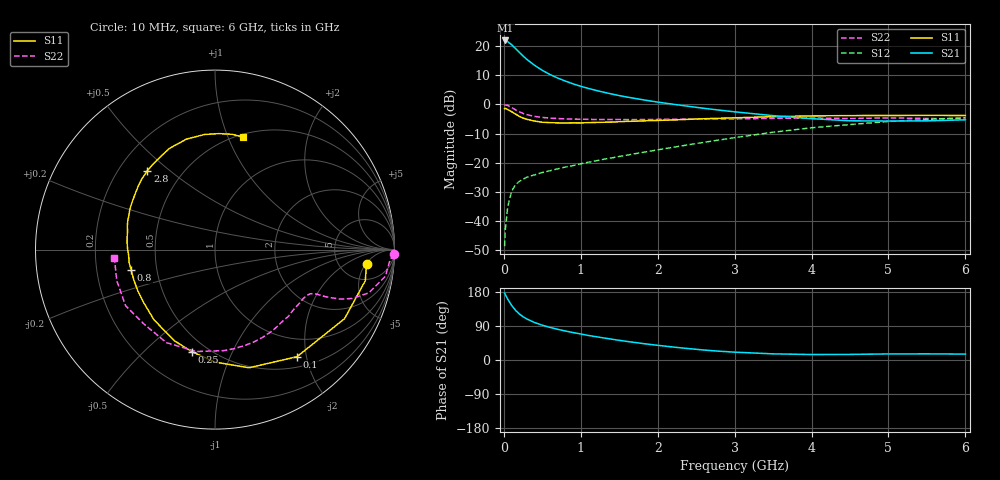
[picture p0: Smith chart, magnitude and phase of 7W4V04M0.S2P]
! Infineon Technologies  Discrete & RF Semiconductors
! BFS17W
! Si NPN RF Bipolar Junction Transistor in SOT323
! VCE = 4 V  IC = 4 mA
! Common Emitter S-Parameters:  August  1999
# GHz  S  MA  R  50
!  f  S11  S21  S12  S22
! GHz  MAG  ANG  MAG  ANG  MAG  ANG  MAG  ANG
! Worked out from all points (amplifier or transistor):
!   36 points, 10 MHz to 6 GHz, reference 50 ohm
!   highest |S21| = 22.0 dB at 20 MHz (marker M1)
!   |S21| within 3 dB of that: start of sweep to 160.8 MHz
!   unconditionally stable (mu >= 1): 623.7 MHz to 2.79 GHz; 4.312 GHz to end of sweep
!   at 250 MHz: K = 0.53, MSG = 21.1 dB, |S12| = -25.6 dB
!   at 1.4 GHz: K = 1.26, MAG = 7.9 dB, |S12| = -18.4 dB
!   at 6 GHz: K = 1.08, MAG = -2.1 dB, |S12| = -4.5 dB
!   S11 on the Smith chart (normalised r, x): 10 MHz: 9, -5; 100 MHz: 0.67, -1.83; 250 MHz: 0.41, -0.71; 800 MHz: 0.36, -0.11; 2.8 GHz: 0.32, +0.42; 6 GHz: 0.53, +1.13
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0.01  0.8485 -5.6  12.51 176.6  0.0037 87.1  0.9965 -1.4
0.02  0.8551 -11.7  12.53 172.1  0.0073 90.6  0.976 -3.7
0.05  0.8179 -28.1  11.97 160.7  0.0174 77.3  0.9611 -8.9
0.1  0.7513 -52.6  10.64 144.6  0.032 65.6  0.8906 -15.7
0.15  0.6852 -73.9  9.169 131.4  0.0418 56.2  0.8113 -19.6
0.2  0.6269 -90.0  7.874 121.7  0.0477 52.4  0.7494 -21.6
0.25  0.583 -102.9  6.773 114.2  0.0522 48.1  0.7008 -22.5
0.3  0.5558 -114.1  5.921 108.2  0.0565 47.3  0.6681 -23.1
0.4  0.5183 -131.0  4.685 98.8  0.062 46.5  0.6226 -23.6
0.5  0.4955 -143.0  3.852 91.8  0.0679 47.5  0.5992 -24.1
0.6  0.4874 -152.2  3.261 86.0  0.073 49.5  0.5834 -25.0
0.8  0.4809 -166.1  2.516 76.5  0.0844 52.5  0.5658 -28.0
0.9  0.4838 -171.5  2.256 72.4  0.0893 54.2  0.5602 -29.7
1.1  0.4875 179.1  1.883 64.7  0.1021 56.7  0.5553 -33.7
1.3  0.4951 171.1  1.619 58.1  0.1148 59.2  0.5504 -38.3
1.6  0.5126 161.4  1.339 49.0  0.1349 61.9  0.5486 -45.5
2.2  0.5417 145.4  1.008 34.2  0.184 65.8  0.5564 -61.7
2.8  0.5791 130.5  0.8 23.2  0.2454 65.7  0.5621 -79.3
3.5  0.618 114.5  0.642 16.2  0.3337 61.8  0.5776 -100.5
4.5  0.6441 95.2  0.524 14.8  0.452 50.0  0.5732 -133.3
5.5  0.6496 81.4  0.523 16.2  0.5533 37.2  0.5739 -162.6
6  0.6459 76.2  0.545 15.6  0.5928 31.0  0.5622 -175.5
